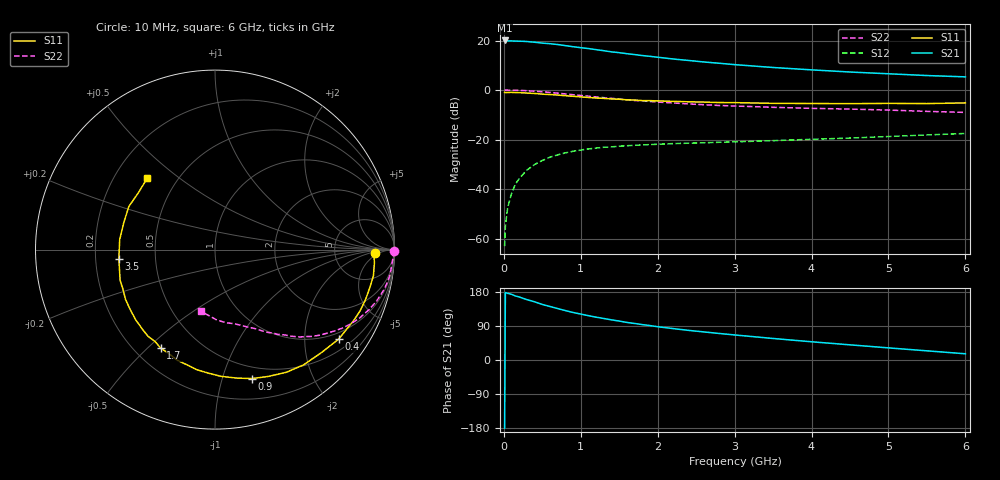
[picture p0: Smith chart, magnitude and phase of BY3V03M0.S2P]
! SIEMENS Small Signal Semiconductors
! BFY420
! Si NPN RF SIEGET Grounded Emitter Transistor in MICRO-X
! VCE = 3 V  IC = 3 mA
! Common Emitter S-Parameters:  October  1996
# GHz  S  MA  R  50
!  f  S11  S21  S12  S22
! GHz  MAG  ANG  MAG  ANG  MAG  ANG  MAG  ANG
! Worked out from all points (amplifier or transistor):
!   36 points, 10 MHz to 6 GHz, reference 50 ohm
!   highest |S21| = 20.0 dB at 10 MHz (marker M1)
!   |S21| within 3 dB of that: start of sweep to 1.023 GHz
!   unconditionally stable (mu >= 1): 3.616 GHz to end of sweep
!   at 250 MHz: K = 0.06, MSG = 26.9 dB, |S12| = -34.0 dB
!   at 1.4 GHz: K = 0.38, MSG = 19.2 dB, |S12| = -23.0 dB
!   at 6 GHz: K = 1.18, MAG = 8.9 dB, |S12| = -17.6 dB
!   S11 on the Smith chart (normalised r, x): 10 MHz: 17, -3; 400 MHz: 0.80, -2.89; 900 MHz: 0.38, -1.25; 1.7 GHz: 0.30, -0.55; 3.5 GHz: 0.30, -0.04; 6 GHz: 0.34, +0.39
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0.01  0.8922 -1.1  10.03 -179.9  0.0007 82.6  0.9957 -0.4
0.02  0.8852 -1.8  9.979 178.1  0.0018 72.4  0.995 -0.9
0.05  0.8913 -4.7  9.801 175.9  0.0042 81.9  0.9943 -2.2
0.1  0.8946 -9.4  9.808 173.4  0.0081 83.5  0.9889 -4.5
0.15  0.8885 -13.5  9.732 168.9  0.0125 80.2  0.9862 -6.9
0.2  0.8838 -18.2  9.674 166.4  0.0162 79.8  0.9829 -8.9
0.3  0.868 -27.1  9.532 159.3  0.0241 74.3  0.9676 -13.4
0.4  0.8505 -35.9  9.234 153.6  0.0313 70.3  0.9454 -17.6
0.5  0.8249 -44.2  8.87 146.6  0.0377 66.1  0.9203 -21.4
0.6  0.8098 -52.5  8.624 141.2  0.044 61.8  0.893 -25.1
0.7  0.7908 -59.8  8.291 135.7  0.049 58.4  0.8638 -28.5
0.9  0.7475 -74.0  7.496 125.4  0.0578 51.2  0.8038 -34.4
1.1  0.7067 -87.4  6.882 117.0  0.0645 46.1  0.7496 -39.6
1.4  0.6603 -103.9  5.901 105.9  0.0709 40.0  0.679 -45.8
1.7  0.6268 -118.8  5.196 96.4  0.0764 35.5  0.6146 -50.7
2  0.6021 -131.5  4.596 87.8  0.0802 32.2  0.5705 -54.8
2.2  0.59 -138.6  4.233 82.9  0.0826 30.5  0.5478 -57.4
2.8  0.5583 -156.8  3.47 70.0  0.088 27.4  0.4868 -64.0
3.5  0.5381 -174.7  2.851 56.8  0.0949 25.7  0.4468 -70.8
4.5  0.53 163.5  2.309 40.0  0.107 23.3  0.4119 -81.4
5.5  0.5319 142.9  1.96 24.2  0.1237 20.7  0.3702 -95.0
6  0.5489 133.4  1.843 16.4  0.1324 18.7  0.3528 -103.0
